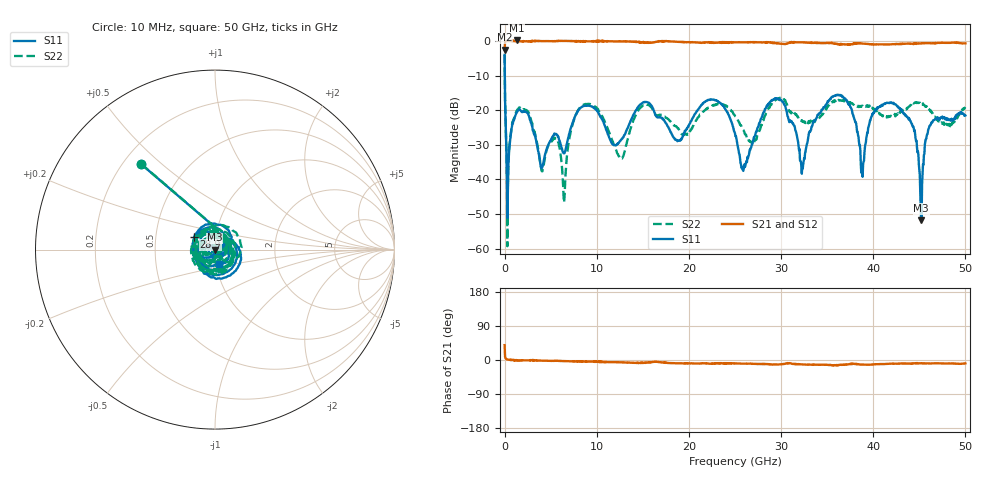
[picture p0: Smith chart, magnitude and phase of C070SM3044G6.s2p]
! 5/19/2020 2:01:04 PM
! D:\C070SM3044G6.S2P
! CHANNEL.1
! TR.MEASUREMENT
! CORRECTED.DATA
# GHZ S RI R 50.0
! FREQ.GHZ  S11RE  S11IM  S21RE  S21IM  S12RE  S12IM  S22RE  S22IM
!; PortSelection: Port_12
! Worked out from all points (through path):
!   1001 points, 10 MHz to 50 GHz, reference 50 ohm
!   highest |S21| = 0.13 dB at 1.31 GHz (marker M1); lowest = -2.5 dB at 10 MHz (marker M2)
!   lowest |S11| = -51.8 dB at 45.2 GHz (marker M3), VSWR 1.01, Z = 49.7 + j0.0177 ohm
!   |S11| at or under -10 dB: 32.87 MHz to end of sweep
!   |S22| runs from -59.3 to -4.0 dB; largest |S21 - S12| = 0.039
!   S11 on the Smith chart (normalised r, x): 10 MHz: 0.27, +0.43; 28.9 GHz: 0.79, +0.11; 50 GHz: 1.03, -0.17
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0.01  -0.4104 0.4753  0.578 0.4716  0.5782 0.4726  -0.4104 0.4764
0.40992  -0.00921 -0.0112  0.998 0.0168  0.9984 0.0171  -0.00857 -0.013
1.30974  -0.0876 0.0302  1.015 -0.0209  1.005 -0.0335  -0.0917 0.0335
4.0092  -0.00674 -0.0128  0.9909 -0.0303  0.9926 -0.0294  -0.00622 -0.0121
5.60888  0.0314 0.0328  0.9966 -0.0413  0.9966 -0.0359  0.0383 0.00959
6.45871  0.0198 0.013  0.9977 -0.0506  0.9972 -0.0504  -0.00408 -0.00221
8.35833  0.0851 -0.0703  0.9844 -0.052  0.9888 -0.0611  0.0902 -0.0709
12.60748  0.0143 -0.0338  0.9756 -0.1035  0.9807 -0.1003  0.0117 -0.0159
16.70666  0.0585 0.052  0.9766 -0.0854  0.9834 -0.0875  0.0797 0.0273
22.65547  0.00201 -0.1414  0.9334 -0.1591  0.9145 -0.1435  -0.0213 -0.1145
25.005  -0.0137 0.0441  0.9422 -0.1557  0.9406 -0.1583  0.0522 0.0642
25.95481  0.013 -0.00702  0.9412 -0.1593  0.9405 -0.1585  0.0365 -0.0345
28.90422  -0.116 0.0706  0.9341 -0.1874  0.9311 -0.1971  -0.0506 0.1104
32.30354  -0.0128 -0.00873  0.9332 -0.191  0.9283 -0.1901  -0.0686 0.000259
33.35333  0.00112 0.058  0.9111 -0.198  0.922 -0.1904  0.0199 0.0689
36.60268  0.00362 -0.1618  0.868 -0.1957  0.8776 -0.1822  -0.1005 -0.0928
38.85223  0.00804 0.00734  0.8981 -0.1895  0.8923 -0.1885  0.1149 0.0106
41.70166  -0.127 0.0124  0.8771 -0.1577  0.8783 -0.1597  -0.0511 0.0645
44.25115  0.0425 0.0407  0.8923 -0.1532  0.8972 -0.1497  0.0644 -0.1044
45.20096  -0.00257 0.000178  0.9152 -0.1361  0.9027 -0.146  -0.1019 -0.0638
46.30074  0.00403 0.0659  0.916 -0.1467  0.9166 -0.1369  -0.0178 0.0919
50  0.0208 -0.0812  0.9096 -0.1438  0.9173 -0.141  -0.1056 -0.033
